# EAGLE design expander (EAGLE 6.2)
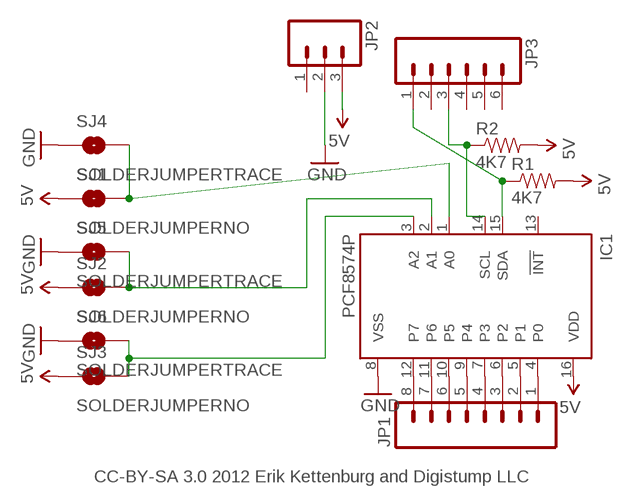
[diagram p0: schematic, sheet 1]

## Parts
IC1  PCF8574P  [DIL16]
JP1  M081X08  [1X08]
JP2  M03PTH  [1X03]
JP3  M06SIP  [1X06]
R1  4K7  RESISTORAXIAL-0.3  [AXIAL-0.3]
R2  4K7  RESISTORAXIAL-0.3  [AXIAL-0.3]
SJ1  SOLDERJUMPERNO  [SJ_2S-NO]
SJ2  SOLDERJUMPERNO  [SJ_2S-NO]
SJ3  SOLDERJUMPERNO  [SJ_2S-NO]
SJ4  SOLDERJUMPERTRACE  [SJ_2S-TRACE]
SJ5  SOLDERJUMPERTRACE  [SJ_2S-TRACE]
SJ6  SOLDERJUMPERTRACE  [SJ_2S-TRACE]

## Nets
5V: IC1.16(VDD) JP2.3 R1.P$2 R2.P$2 SJ1.1 SJ2.1 SJ3.1
GND: IC1.8(VSS) JP2.2 SJ4.1 SJ5.1 SJ6.1
N$1: IC1.14(SCL) JP3.3 R2.P$1
N$2: IC1.15(SDA) JP3.1 R1.P$1
N$3: IC1.1(A0) SJ1.2 SJ4.2
N$4: IC1.2(A1) SJ2.2 SJ5.2
N$5: IC1.3(A2) SJ3.2 SJ6.2
N$6: IC1.4(P0) JP1.1
N$7: IC1.5(P1) JP1.2
N$8: IC1.6(P2) JP1.3
N$9: IC1.7(P3) JP1.4
N$10: IC1.9(P4) JP1.5
N$11: IC1.10(P5) JP1.6
N$12: IC1.11(P6) JP1.7
N$13: IC1.12(P7) JP1.8
Unconnected: IC1.13(!INT) JP2.1 JP3.2 JP3.4 JP3.5 JP3.6

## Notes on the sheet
- CC-BY-SA 3.0 2012 Erik Kettenburg and Digistump LLC

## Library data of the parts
IC1 = micro-philips:PCF8574: I2C-Bus Remote 8-bit I/O expander http://www.semiconductors.philips.com/acrobat_download/datasheets/PCF8574_4.pdf; MPN: PCF8574PN; OC_FARNELL: 204020; OC_NEWARK: 11N8515
JP1 = SparkFun:M08: Header 8 Standard 8-pin 0.1" header. Use with straight break away headers (SKU : PRT-00116), right angle break away headers (PRT-00553), swiss pins (PRT-00743), machine pins (PRT-00117), and female headers (PRT-00115).
JP2 = SparkFun:M03: Header 3 Standard 3-pin 0.1" header. Use with straight break away headers (SKU : PRT-00116), right angle break away headers (PRT-00553), swiss pins (PRT-00743), machine pins (PRT-00117), and female headers (PRT-00115). Molex polarized connector foot print use with SKU : PRT-08232 with associated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
JP3 = SparkFun:M06: Header 6 Standard 6-pin 0.1" header. Use with straight break away headers (SKU : PRT-00116), right angle break away headers (PRT-00553), swiss pins (PRT-00743), machine pins (PRT-00117), and female headers (PRT-00115). Molex polarized connector foot print use with SKU : PRT-08094 with associated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
R1 R2 = SparkFun:RESISTOR: Resistor
SJ1-SJ6 = SparkFun:SOLDERJUMPER: Solder Jumper

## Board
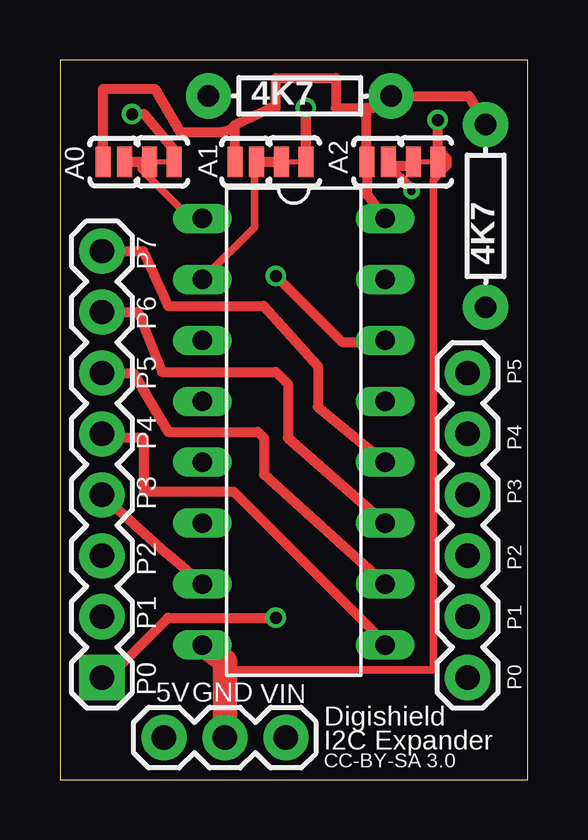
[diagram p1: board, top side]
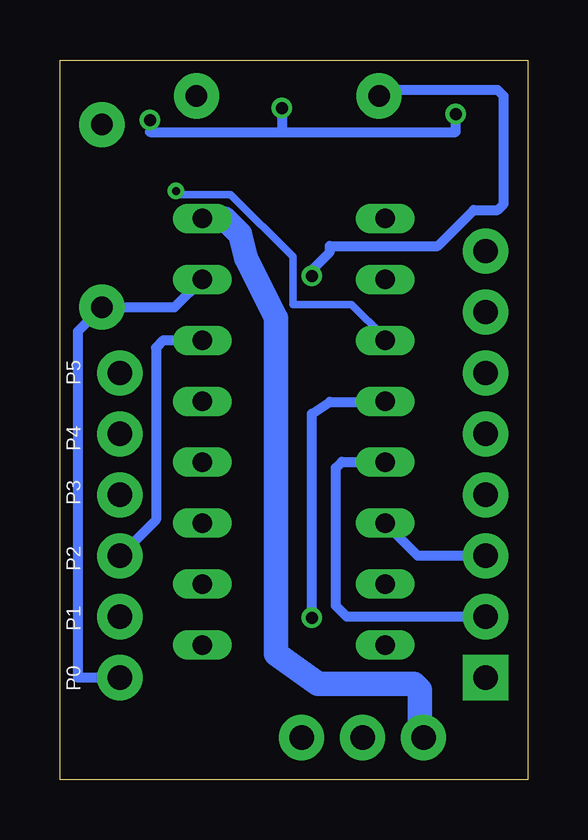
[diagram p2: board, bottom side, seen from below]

Size 19.5 x 30 mm. Coordinates in mm from the lower left corner, seen from the top.
Outline: 0,30 0,0 19.5,0 19.5,30 0,30
Copper layers (1*16): Top 0.0356mm / dielectric 1.5011mm / Bottom 0.0356mm
Design rules: minimum track width 12mil, minimum drill 13mil, track to track 8mil, track to pad 8mil, pad to pad 8mil, via to via 8mil, smd to smd 8mil, copper to edge 15mil, drill to drill 12mil, minimum pad ring 7mil, minimum via ring 7mil, stop-mask expansion 4mil, vias tented up to drill 24mil, thermal gap 10mil

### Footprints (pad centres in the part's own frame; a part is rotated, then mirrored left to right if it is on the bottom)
DIL16 = drill 0.813 long: 1 -8.89,-3.81; 2 -6.35,-3.81; 3 -3.81,-3.81; 4 -1.27,-3.81; 5 1.27,-3.81; 6 3.81,-3.81; 7 6.35,-3.81; 8 8.89,-3.81; 9 8.89,3.81; 10 6.35,3.81; 11 3.81,3.81; 12 1.27,3.81; 13 -1.27,3.81; 14 -3.81,3.81; 15 -6.35,3.81; 16 -8.89,3.81
1X08 = drill 1.016 pad 1.88 square: 1 0,0 | drill 1.016 pad 1.88: 2 2.54,0; 3 5.08,0; 4 7.62,0; 5 10.16,0; 6 12.7,0; 7 15.24,0; 8 17.78,0
1X03 = drill 1.016 pad 1.88: 1 0,0; 2 2.54,0; 3 5.08,0
1X06 = drill 1.016 pad 1.88: 1 0,0; 2 2.54,0; 3 5.08,0; 4 7.62,0; 5 10.16,0; 6 12.7,0
AXIAL-0.3 = drill 0.9 pad 1.88: P$1 -3.81,0; P$2 3.81,0
SJ_2S-NO = smd 0.635 x 1.27: 1 -0.45,0; 2 0.45,0
SJ_2S-TRACE = smd 0.635 x 1.27: 1 -0.508,0; 2 0.508,0

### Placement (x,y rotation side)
IC1  9.75,14.5 270 top
JP1  1.75,4.25 90 top
JP2  9.42,1.75 180 top
JP3  17,4.25 90 top
R1  17.75,23.5 90 top
R2  10,28.5 0 top
SJ1  2.25,25.75 0 top
SJ2  7.75,25.75 0 top
SJ3  13.25,25.75 0 top
SJ4  4.25,25.75 180 top
SJ5  9.75,25.75 180 top
SJ6  15.25,25.75 180 top

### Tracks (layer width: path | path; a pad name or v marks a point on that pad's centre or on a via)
5V
  Top 0.406: R1.P$2 17.06,28.5 R2.P$2 13.06,28 12.75,28 | IC1.16 12.8,24.4 SJ3.1 12.75,25.8 12.75,28 | SJ1.1 1.8,28.8 3.95,28.8 5,27 6.75,27 7.12,27.12 | 7.12,27.12 7.3,27.3 | 7.3,27.2 7.12,27.12 | SJ2.1 7.3,27.2 | 7.3,27.2 7.3,27.3 | 7.3,27.3 8.75,28 9,28 9,29.25 11.5,29.25 11.5,28 12.75,28
  Bottom 1.016: IC1.16 12.64,23.39 12,22.75 11.75,21.75 10.5,19.25 10.5,5.25 8.75,4 4.75,4 4.5,3.75 4.5,1.91 JP2.3
GND  (via drill 0.5)
  Top 0.305: 6.88,4.57 15.58,4.57 15.58,24.99 16.19,25.6 16.19,25.91 15.88,26.21 SJ6.1
  Top 0.406: SJ6.1 15.76,27.24 v15.75,27.5 | v3,27.75 3.5,27.75 4.75,26.25 SJ4.1 | v10.25,28 SJ5.1 10.26,27.24 v10.25,28
  Top 1.016: JP2.2 6.88,4.57 6.88,4.92 IC1.8
  Bottom 0.406: v15.75,27.5 15.75,27 10.25,27 | v10.25,28 10.25,27 | 10.25,27 3,27 v3,27.75
N$1  (via drill 0.5)
  Top 0.406: v9,21 11.75,18.25 13.5,18.25 IC1.14
  Bottom 0.406: JP3.3 15.5,10.83 15.5,18 15.19,18.31 IC1.14 | v9,21 9,21.25 8.25,22 8.25,22.25 3.75,22.25 2.25,23.75 1.25,23.75 1,24 1,28.5 1.25,28.75 5.69,28.75 R2.P$1
N$2
  Bottom 0.406: JP3.1 18.75,4.25 18.75,18.69 R1.P$1 14.72,19.69 IC1.15
N$3
  Top 0.305: 3.38,25.75 3.38,25.45 5.37,23.47 5.82,23.47 IC1.1
  Top 0.406: SJ4.2 3.38,25.75 SJ1.2
N$4
  Top 0.305: SJ2.2 8.11,25.6 8.11,23.01 5.97,20.88 IC1.2
  Top 0.406: SJ5.2 SJ2.2
N$5  (via drill 0.33)
  Top 0.305: v14.66,24.54 14.66,24.69 13.75,25.6 SJ3.2
  Top 0.406: 13.75,25.6 14.6,25.6 SJ6.2
  Bottom 0.305: v14.66,24.54 14.51,24.38 12.38,24.38 9.78,21.79 9.78,19.81 7.35,19.81 5.97,18.44 IC1.3
N$6  (via drill 0.5)
  Top 0.406: JP1.1 2,4.25 4.5,6.75 v9,6.75
  Bottom 0.406: v9,6.75 9,15.25 8.25,15.75 5.96,15.75 IC1.4
N$7
  Bottom 0.406: JP1.2 7.54,6.79 8,7.25 8,13 7.75,13.25 5.96,13.25 IC1.5
N$8
  Bottom 0.406: JP1.3 4.58,9.33 IC1.6
N$9
  Top 0.406: IC1.7 4.44,9.43 JP1.4
N$10
  Top 0.406: IC1.9 13.31,5.94 7.25,12 3.5,12 3.5,14.25 1.91,14.25 JP1.5
N$11
  Top 0.406: JP1.6 3.05,16.95 4.5,14.5 8.25,14.5 8.5,14.25 8.5,12.71 IC1.10
N$12
  Top 0.406: JP1.7 3.26,19.49 4.25,17 9,17 9.5,16.5 9.5,14.25 IC1.11
N$13
  Top 0.406: JP1.8 3.47,22.03 4.5,19.75 8.5,19.75 10.75,17.25 10.75,15.54 IC1.12

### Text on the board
tPlace: A1 | A0 | A2 | P7 | P6 | P5 | P4 | P3 | P2 | P1 | P0 | VIN | 5V | GND | Digishield | I2C Expander | CC-BY-SA 3.0
tNames: P5 | P4 | P3 | P2 | P1 | P0
bNames: P5 | P4 | P3 | P2 | P1 | P0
